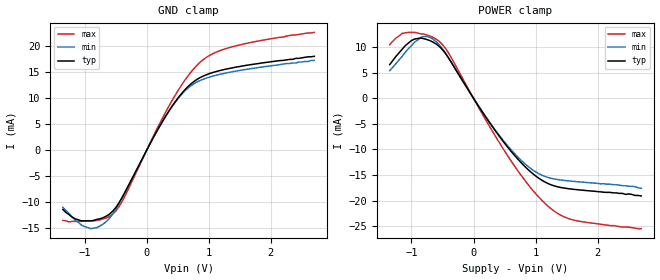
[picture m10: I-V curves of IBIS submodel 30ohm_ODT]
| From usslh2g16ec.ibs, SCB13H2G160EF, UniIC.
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| SUBMODEL 30ohm_ODT
[Submodel]   30ohm_ODT
Submodel_type  Dynamic_clamp
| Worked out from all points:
|   GND clamp passes 1 mA (typ) near -0.04 V on its own axis
|   POWER clamp passes 1 mA (typ) near -0.05 V on its own axis
[GND Clamp]
|Voltage   I(typ)   I(min)   I(max)
-1.35V    -11.4mA    -11mA      -13.5mA
-1.15V    -13.2mA    -13.5mA    -13.7mA
-900mV    -13.6mA    -15.1mA    -13.6mA
-650mV    -12.69mA   -13.72mA   -13.05mA
-500mV    -11.08mA   -11.45mA   -11.74mA
-400mV    -9.181mA   -9.306mA   -9.948mA
100mV     2.276mA    2.274mA    2.513mA
400mV     8.316mA    8.244mA    9.382mA
650mV     12.08mA    11.81mA    14.07mA
900mV     14.23mA    13.63mA    17.35mA
1.45V     16.04mA    15.27mA    20.16mA
2.7V      18.1mA     17.3mA     22.7mA
[POWER Clamp]
|Voltage   I(typ)   I(min)   I(max)
-1.35V    6.6mA      5.4mA      10.5mA
-1.15V    9.6mA      8.2mA      12.7mA
-1V       11.3mA     10.3mA     12.9mA
-850mV    11.8mA     11.9mA     12.6mA
-700mV    11.28mA    11.9mA     12.18mA
-400mV    7.848mA    7.858mA    8.822mA
150mV     -2.816mA   -2.766mA   -3.241mA
550mV     -9.562mA   -9.285mA   -11.25mA
900mV     -14.18mA   -13.52mA   -17.19mA
1.2V      -16.67mA   -15.49mA   -21.11mA
1.6V      -17.79mA   -16.23mA   -23.78mA
2.7V      -19.1mA    -17.6mA    -25.5mA
